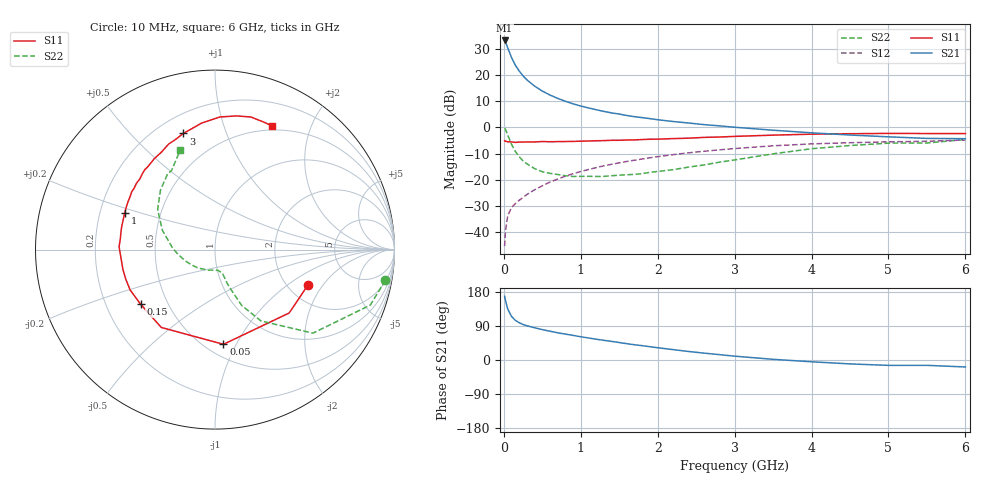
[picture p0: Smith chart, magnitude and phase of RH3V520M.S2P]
! SIEMENS Small Signal Semiconductors
! BFR106
! Si NPN RF Bipolar Junction Transistor in SOT23
! VCE = 3.5 V  IC = 20 mA
! Common Emitter S-Parameters:  August  1996
# GHz  S  MA  R  50
!  f  S11  S21  S12  S22
! GHz  MAG  ANG  MAG  ANG  MAG  ANG  MAG  ANG
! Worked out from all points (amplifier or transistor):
!   36 points, 10 MHz to 6 GHz, reference 50 ohm
!   highest |S21| = 33.1 dB at 10 MHz (marker M1)
!   |S21| within 3 dB of that: start of sweep to 53.09 MHz
!   unconditionally stable (mu >= 1): 370 MHz to 2.249 GHz; 5.419 GHz to end of sweep
!   at 250 MHz: K = 0.89, MSG = 23.2 dB, |S12| = -26.7 dB
!   at 1.4 GHz: K = 1.07, MAG = 8.2 dB, |S12| = -14.1 dB
!   at 6 GHz: K = 1.00, MAG = -0.1 dB, |S12| = -4.8 dB
!   S11 on the Smith chart (normalised r, x): 10 MHz: 2.56, -1.45; 50 MHz: 0.61, -0.89; 150 MHz: 0.35, -0.29; 1 GHz: 0.31, +0.18; 3 GHz: 0.31, +0.72; 6 GHz: 0.45, +1.47
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0.01  0.5542 -20.8  45.38 168.1  0.0054 83.8  0.965 -10.2
0.02  0.5436 -40.5  42.93 158.2  0.0102 76.5  0.9184 -19.7
0.05  0.5298 -84.9  32.99 134.9  0.0204 60.2  0.7169 -40.5
0.1  0.527 -124.6  21.5 115.0  0.0296 53.7  0.4728 -57.2
0.15  0.5143 -143.8  15.26 104.5  0.035 53.2  0.3457 -64.4
0.2  0.5236 -154.6  11.85 98.4  0.0405 55.3  0.2753 -66.6
0.25  0.5238 -161.9  9.56 93.7  0.046 57.8  0.2274 -68.9
0.3  0.5247 -167.7  8.033 90.4  0.0523 60.2  0.201 -70.1
0.4  0.5265 -175.5  6.113 85.1  0.0642 63.0  0.1629 -71.3
0.5  0.5346 178.4  4.91 80.2  0.0767 64.6  0.1422 -72.3
0.6  0.5308 173.3  4.126 75.9  0.0901 65.6  0.1323 -74.3
0.7  0.5332 169.3  3.57 71.8  0.1031 65.8  0.1257 -77.4
0.8  0.5357 165.5  3.138 68.3  0.1167 65.6  0.1192 -80.4
1  0.5433 157.7  2.547 61.4  0.1435 64.5  0.1161 -86.6
1.1  0.548 154.4  2.342 58.1  0.1565 63.9  0.1162 -91.8
1.6  0.5727 139.8  1.676 43.0  0.2234 58.5  0.1243 -115.9
2.2  0.6089 123.8  1.29 27.4  0.3007 50.5  0.1555 -146.6
3  0.6707 105.3  1.003 10.1  0.3937 38.4  0.2386 177.1
3.5  0.7089 96.0  0.88 1.8  0.444 30.7  0.3121 159.9
4.5  0.7543 80.9  0.712 -10.3  0.5079 15.2  0.4491 132.6
5.5  0.7607 69.2  0.614 -14.1  0.5424 5.1  0.5014 119.0
6  0.759 65.2  0.606 -18.4  0.5726 -2.3  0.5854 109.4
